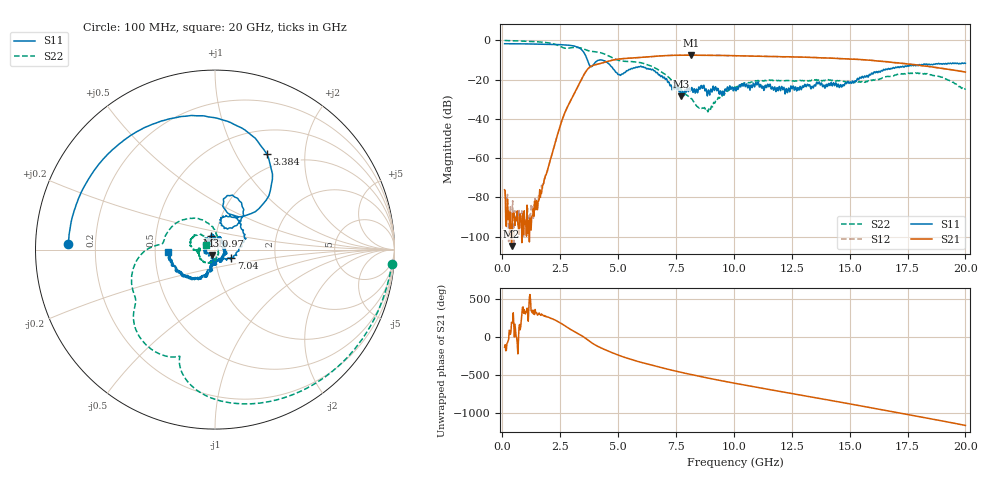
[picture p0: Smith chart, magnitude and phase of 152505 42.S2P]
!  2-Port S-parameters saved by WinCal
! VAR MeasName=S-Parameters (CALIBRATED_DATA) read from VNA (N5230C)
! VAR MeasDate=4/10/2015 9:32:39 AM
! VAR NAME=152505 42
! VAR FILENAME=152505 42.S2P
! VAR DATE=4/10/2015 9:32:40 AM
! VAR PHYS_PORTS=1,2
# Hz S DB R 50
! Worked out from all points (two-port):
!   801 points, 100 MHz to 20 GHz, reference 50 ohm
!   highest |S21| = -7.55 dB at 8.135 GHz (marker M1); lowest = -104.8 dB at 398.5 MHz (marker M2)
!   |S21| within 3 dB of the highest: 4.612 GHz to 16.22 GHz (11.6 GHz wide, 111 % of centre)
!   lowest |S11| = -28.6 dB at 7.737 GHz (marker M3), VSWR 1.08, Z = 48 - j3.08 ohm
!   |S11| at or under -10 dB: 3.675 GHz to 4.207 GHz (532.4 MHz wide, 13.5 % of centre); 4.253 GHz to end of sweep
!   |S22| runs from -36.4 to -0.1 dB; largest |S21 - S12| = 0.0058
!   S11 on the Smith chart (normalised r, x): 100 MHz: 0.10, +0.02; 3.384 GHz: 0.80, +1.35; 7.04 GHz: 1.19, -0.11; 10.97 GHz: 0.95, +0.15; 20 GHz: 0.59, -0.02
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1e8  -1.75 177.6  -76.13 -136.0  -76.44 -17.6  -0.08 -4.6
3.985e8  -1.77 170.5  -104.77 -170.4  -88.17 -110.0  -0.22 -16.5
1.617375e9  -1.93 140.1  -76.01 -66.2  -77.78 -64.9  -0.84 -66.1
2.612375e9  -2.28 107.9  -39.60 160.4  -39.68 160.6  -3.73 -107.8
3.3835e9  -4.35 61.5  -20.74 23.0  -20.75 23.4  -3.90 -132.0
3.43325e9  -4.88 57.6  -19.59 13.9  -19.59 14.2  -4.05 -134.6
3.9805e9  -11.84 79.7  -12.57 -102.2  -12.57 -101.8  -5.80 -152.0
4.62725e9  -12.21 49.9  -10.51 165.7  -10.51 165.9  -8.12 -178.7
5.448125e9  -15.11 78.6  -9.14 73.7  -9.10 73.7  -10.82 169.0
6.741625e9  -17.54 2.4  -8.02 -34.5  -8.02 -34.6  -15.08 112.3
7.040125e9  -19.94 -26.8  -7.82 -57.0  -7.82 -56.9  -17.37 98.9
7.736625e9  -28.56 -121.0  -7.59 -107.1  -7.58 -106.8  -25.23 75.5
8.134625e9  -25.66 -172.9  -7.55 -133.4  -7.57 -133.4  -29.41 64.6
8.880875e9  -26.30 135.6  -7.62 179.3  -7.63 179.4  -36.40 -7.8
1.005e10  -24.06 146.9  -7.83 110.6  -7.86 110.4  -23.88 -97.9
1.097038e10  -21.89 104.5  -8.10 59.6  -8.06 59.5  -20.62 -131.0
1.216438e10  -23.95 21.0  -8.39 -4.4  -8.38 -4.4  -20.57 -159.3
1.338325e10  -23.38 -76.7  -8.76 -70.4  -8.70 -70.1  -20.28 -168.4
1.51245e10  -20.79 -100.2  -9.62 -164.7  -9.62 -164.8  -21.44 177.9
1.669162e10  -14.37 -118.7  -11.04 107.9  -10.99 107.2  -18.47 -179.8
1.83085e10  -12.08 -152.4  -13.23 17.8  -13.04 17.0  -17.15 144.6
2e10  -11.71 -176.5  -16.16 -80.8  -16.19 -80.9  -25.13 152.9
